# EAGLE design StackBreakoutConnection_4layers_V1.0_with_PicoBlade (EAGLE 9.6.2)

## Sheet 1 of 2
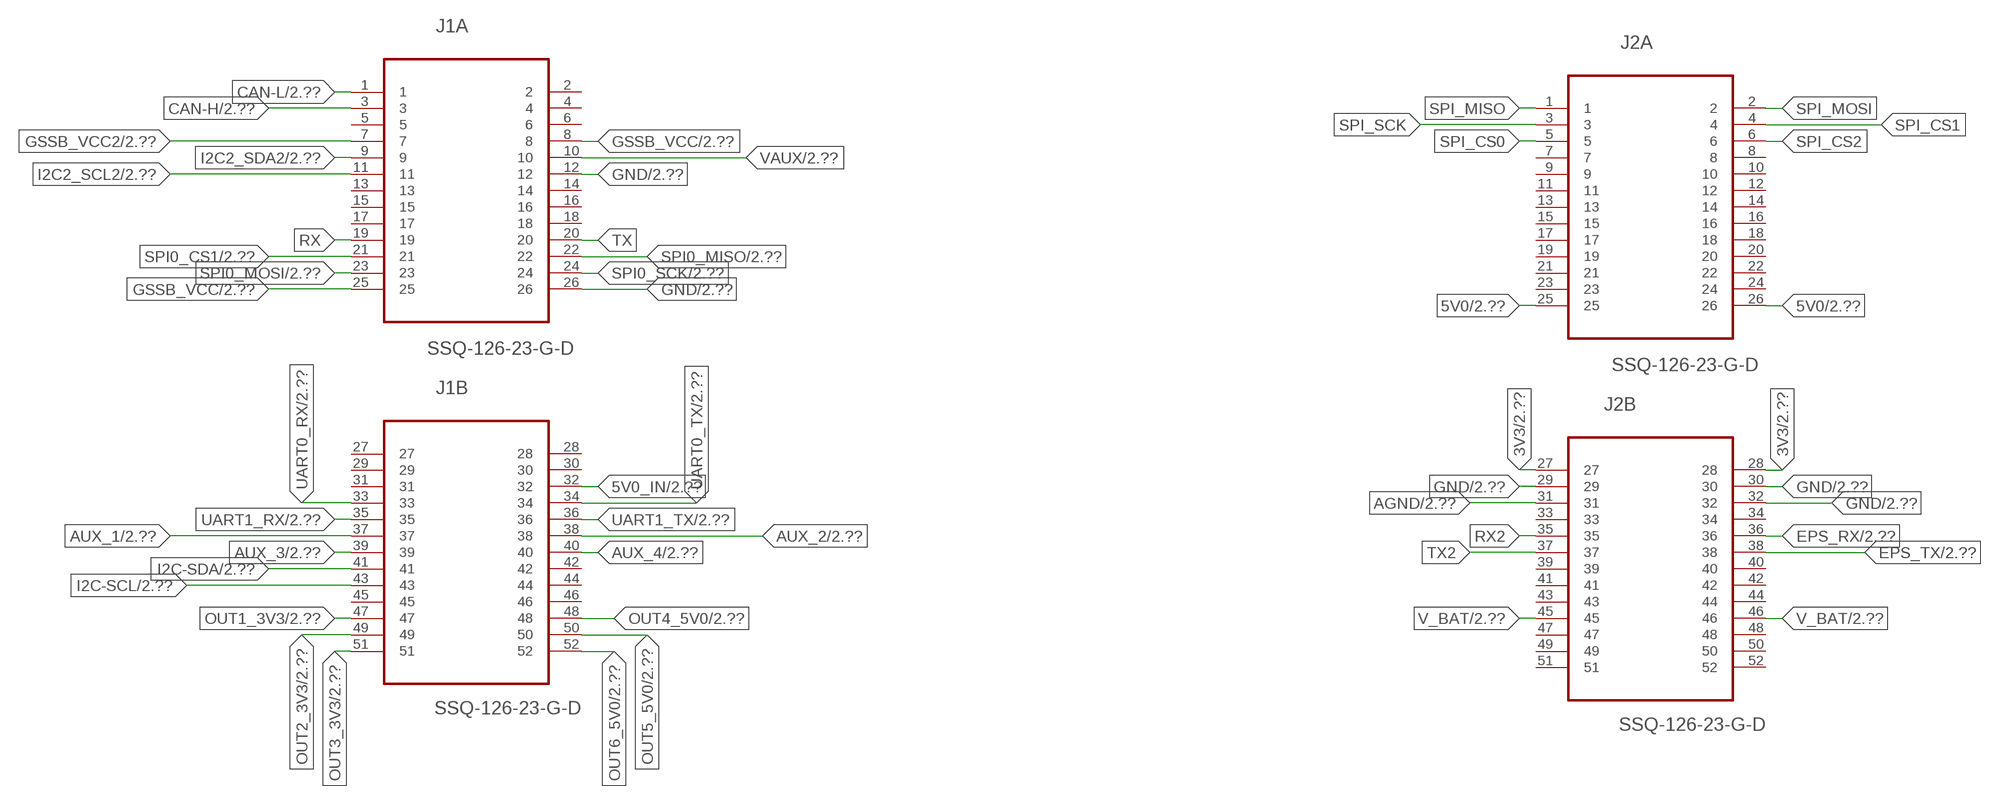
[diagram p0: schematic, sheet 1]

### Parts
J1  SSQ-126-23-G-D  [SAMTEC_SSQ-126-23-G-D]
J2  SSQ-126-23-G-D  [SAMTEC_SSQ-126-23-G-D]

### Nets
3V3: J2.27 J2.28 ; also sheet 2
5V0: J2.25 J2.26 ; also sheet 2
5V0_IN: J1.32 ; also sheet 2
AGND: J2.31 ; also sheet 2
AUX_1: J1.37 ; also sheet 2
AUX_2: J1.38 ; also sheet 2
AUX_3: J1.39 ; also sheet 2
AUX_4: J1.40 ; also sheet 2
CAN-H: J1.3 ; also sheet 2
CAN-L: J1.1 ; also sheet 2
EPS_RX: J2.36 ; also sheet 2
EPS_TX: J2.38 ; also sheet 2
GND: J1.12 J1.26 J2.29 J2.30 J2.32 ; also sheet 2
GSSB_VCC: J1.8 J1.25 ; also sheet 2
GSSB_VCC2: J1.7 ; also sheet 2
I2C2_SCL2: J1.11 ; also sheet 2
I2C2_SDA2: J1.9 ; also sheet 2
I2C-SCL: J1.43 ; also sheet 2
I2C-SDA: J1.41 ; also sheet 2
OUT1_3V3: J1.47 ; also sheet 2
OUT2_3V3: J1.49 ; also sheet 2
OUT3_3V3: J1.51 ; also sheet 2
OUT4_5V0: J1.48 ; also sheet 2
OUT5_5V0: J1.50 ; also sheet 2
OUT6_5V0: J1.52 ; also sheet 2
RX: J1.19
RX2: J2.35
SPI0_CS1: J1.21 ; also sheet 2
SPI0_MISO: J1.22 ; also sheet 2
SPI0_MOSI: J1.23 ; also sheet 2
SPI0_SCK: J1.24 ; also sheet 2
SPI_CS0: J2.5
SPI_CS1: J2.4
SPI_CS2: J2.6
SPI_MISO: J2.1
SPI_MOSI: J2.2
SPI_SCK: J2.3
TX: J1.20
TX2: J2.37
UART0_RX: J1.33 ; also sheet 2
UART0_TX: J1.34 ; also sheet 2
UART1_RX: J1.35 ; also sheet 2
UART1_TX: J1.36 ; also sheet 2
V_BAT: J2.45 J2.46 ; also sheet 2
VAUX: J1.10 ; also sheet 2
Unconnected: J1.2 J1.4 J1.5 J1.6 J1.13 J1.14 J1.15 J1.16 J1.17 J1.18 J1.27 J1.28 J1.29 J1.30 J1.31 J1.42 J1.44 J1.45 J1.46 J2.7 J2.8 J2.9 J2.10 J2.11 J2.12 J2.13 J2.14 J2.15 J2.16 J2.17 J2.18 J2.19 J2.20 J2.21 J2.22 J2.23 J2.24 J2.33 J2.34 J2.39 J2.40 J2.41 J2.42 J2.43 J2.44 J2.47 J2.48 J2.49 J2.50 J2.51 J2.52

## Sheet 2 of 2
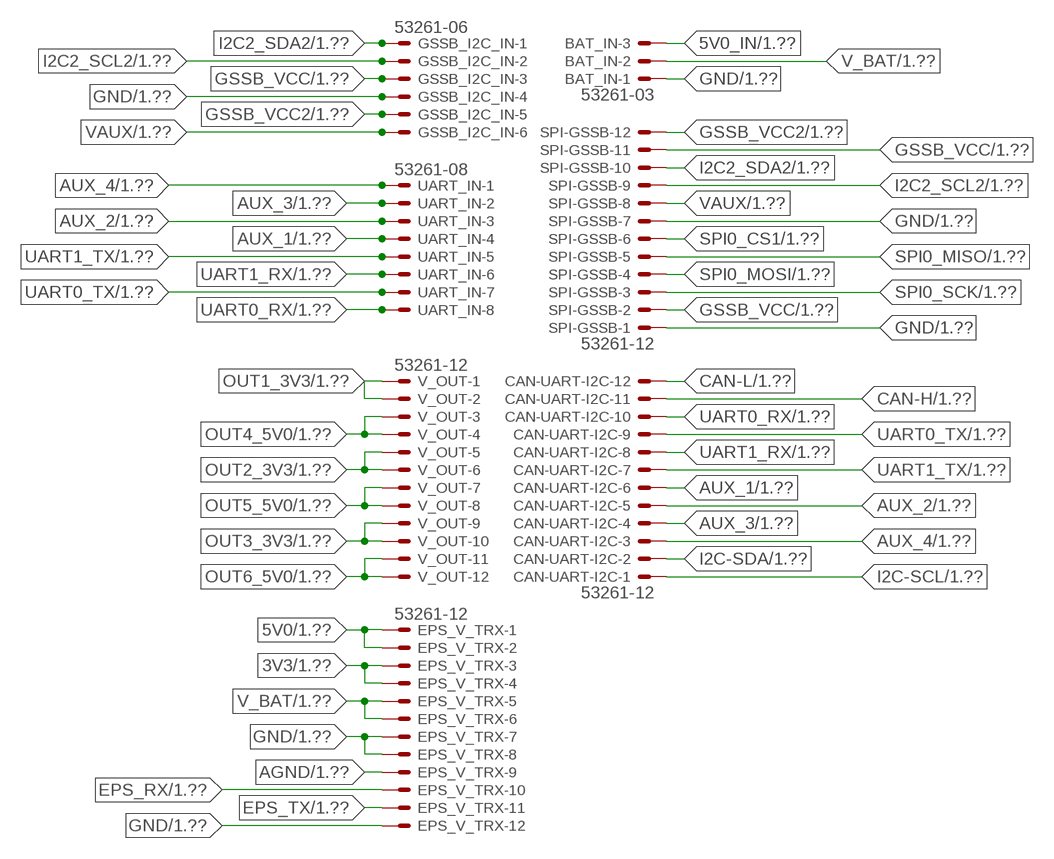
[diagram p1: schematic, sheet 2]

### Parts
BAT_IN  53261-03  [53261-03]
CAN-UART-I2C  53261-12  [53261-12]
EPS_V_TRX  53261-12  [53261-12]
GSSB_I2C_IN  53261-06  [53261-06]
SPI-GSSB  53261-12  [53261-12]
UART_IN  53261-08  [53261-08]
V_OUT  53261-12  [53261-12]

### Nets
3V3: EPS_V_TRX.3 EPS_V_TRX.4 ; also sheet 1
5V0: EPS_V_TRX.1 EPS_V_TRX.2 ; also sheet 1
5V0_IN: BAT_IN.3 ; also sheet 1
AGND: EPS_V_TRX.9 ; also sheet 1
AUX_1: CAN-UART-I2C.6 UART_IN.4 ; also sheet 1
AUX_2: CAN-UART-I2C.5 UART_IN.3 ; also sheet 1
AUX_3: CAN-UART-I2C.4 UART_IN.2 ; also sheet 1
AUX_4: CAN-UART-I2C.3 UART_IN.1 ; also sheet 1
CAN-H: CAN-UART-I2C.11 ; also sheet 1
CAN-L: CAN-UART-I2C.12 ; also sheet 1
EPS_RX: EPS_V_TRX.10 ; also sheet 1
EPS_TX: EPS_V_TRX.11 ; also sheet 1
GND: BAT_IN.1 EPS_V_TRX.7 EPS_V_TRX.8 EPS_V_TRX.12 GSSB_I2C_IN.4 SPI-GSSB.1 SPI-GSSB.7 ; also sheet 1
GSSB_VCC: GSSB_I2C_IN.3 SPI-GSSB.2 SPI-GSSB.11 ; also sheet 1
GSSB_VCC2: GSSB_I2C_IN.5 SPI-GSSB.12 ; also sheet 1
I2C2_SCL2: GSSB_I2C_IN.2 SPI-GSSB.9 ; also sheet 1
I2C2_SDA2: GSSB_I2C_IN.1 SPI-GSSB.10 ; also sheet 1
I2C-SCL: CAN-UART-I2C.1 ; also sheet 1
I2C-SDA: CAN-UART-I2C.2 ; also sheet 1
OUT1_3V3: V_OUT.1 V_OUT.2 ; also sheet 1
OUT2_3V3: V_OUT.5 V_OUT.6 ; also sheet 1
OUT3_3V3: V_OUT.9 V_OUT.10 ; also sheet 1
OUT4_5V0: V_OUT.3 V_OUT.4 ; also sheet 1
OUT5_5V0: V_OUT.7 V_OUT.8 ; also sheet 1
OUT6_5V0: V_OUT.11 V_OUT.12 ; also sheet 1
SPI0_CS1: SPI-GSSB.6 ; also sheet 1
SPI0_MISO: SPI-GSSB.5 ; also sheet 1
SPI0_MOSI: SPI-GSSB.4 ; also sheet 1
SPI0_SCK: SPI-GSSB.3 ; also sheet 1
UART0_RX: CAN-UART-I2C.10 UART_IN.8 ; also sheet 1
UART0_TX: CAN-UART-I2C.9 UART_IN.7 ; also sheet 1
UART1_RX: CAN-UART-I2C.8 UART_IN.6 ; also sheet 1
UART1_TX: CAN-UART-I2C.7 UART_IN.5 ; also sheet 1
V_BAT: BAT_IN.2 EPS_V_TRX.5 EPS_V_TRX.6 ; also sheet 1
VAUX: GSSB_I2C_IN.6 SPI-GSSB.8 ; also sheet 1

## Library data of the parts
BAT_IN = con-molex:53?-03: CONNECTOR wire to board 1.25 mm (.049 inch) pitch header; MF: MOLEX; MPN: 53261-0390; OC_FARNELL: 1125359; OC_NEWARK: 57H5006
CAN-UART-I2C EPS_V_TRX SPI-GSSB V_OUT = con-molex:53?-12: CONNECTOR wire to board 1.25 mm (.049 inch) pitch header; MF: MOLEX; MPN: 53261-1271; OC_FARNELL: 1125363; OC_NEWARK: 59J0244
GSSB_I2C_IN = con-molex:53?-06: CONNECTOR wire to board 1.25 mm (.049 inch) pitch header; MF: MOLEX; OC_FARNELL: 1125375; OC_NEWARK: unknown
J1 J2 = SPEL:SSQ-126-23-G-D: CONN RECEPTACLE, 2.54MM, DUAL, 52WAY; MPN: SSQ-126-23-G-D; OC_FARNELL: -; OC_NEWARK: 82P0504; PACKAGE: RECEPTACLE, 2.54MM, DUAL, 52WAY; SUPPLIER: Samtec
UART_IN = con-molex:53?-08: CONNECTOR wire to board 1.25 mm (.049 inch) pitch header; MF: MOLEX; OC_FARNELL: 1125376; OC_NEWARK: unknown

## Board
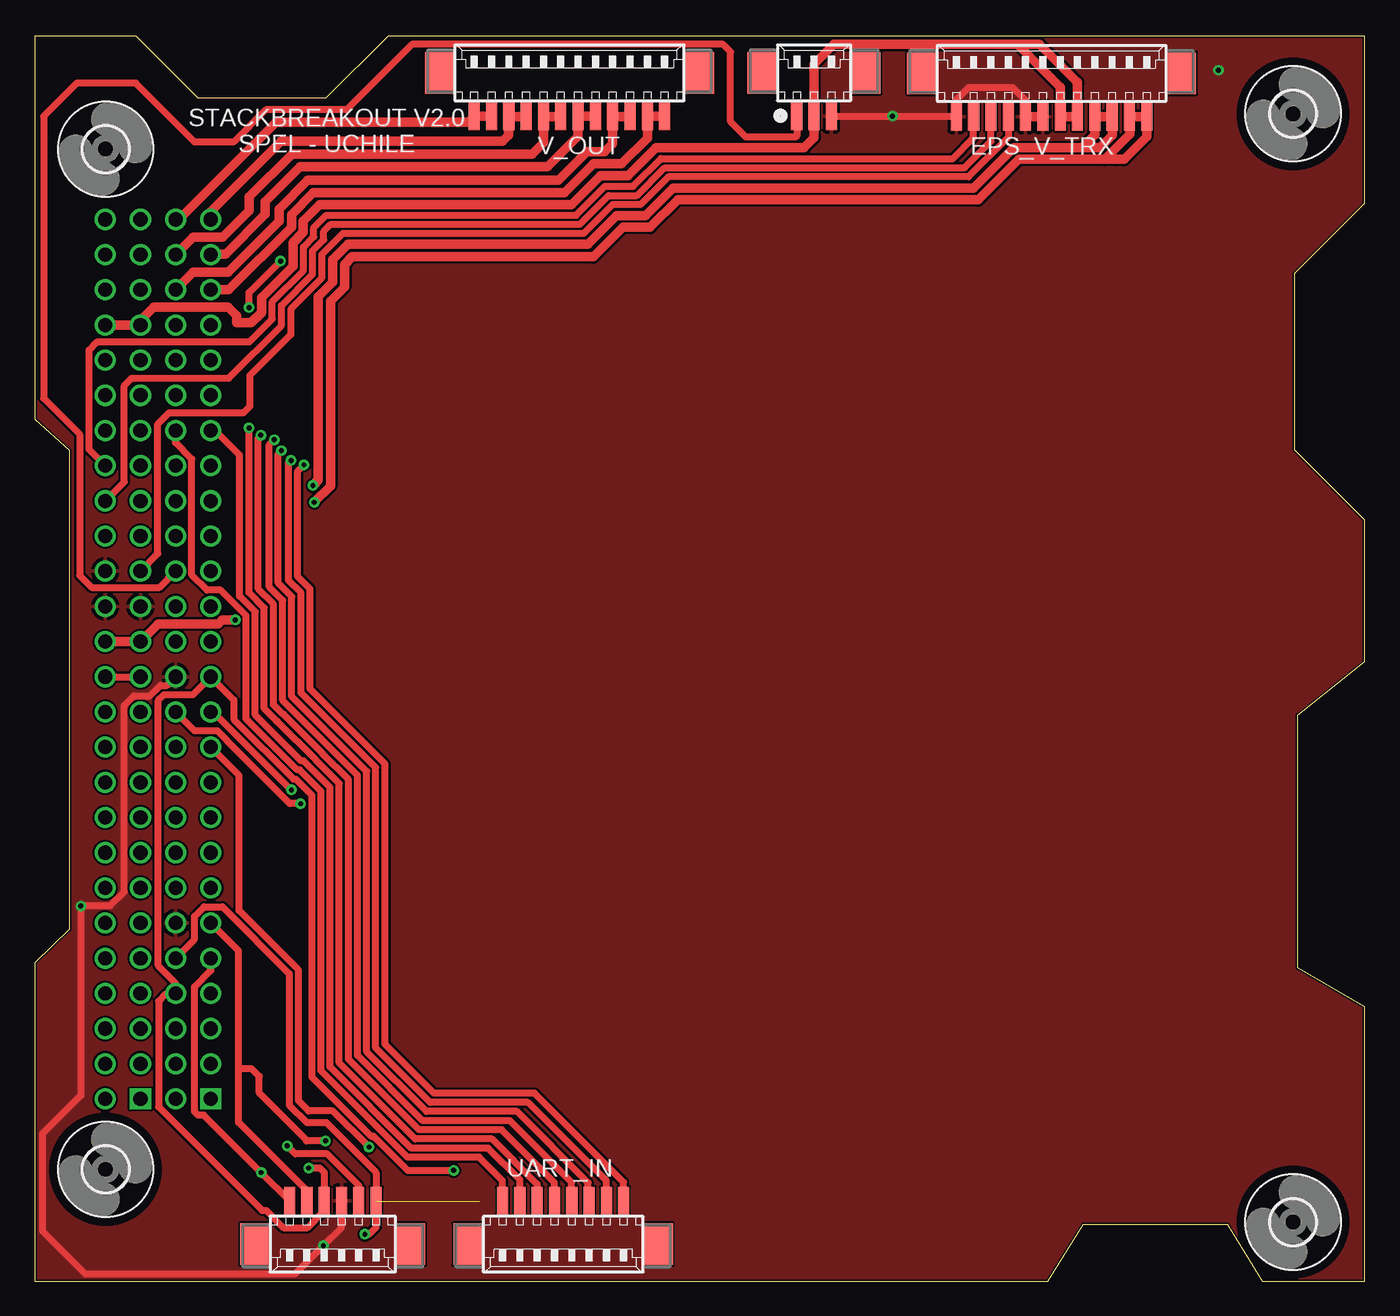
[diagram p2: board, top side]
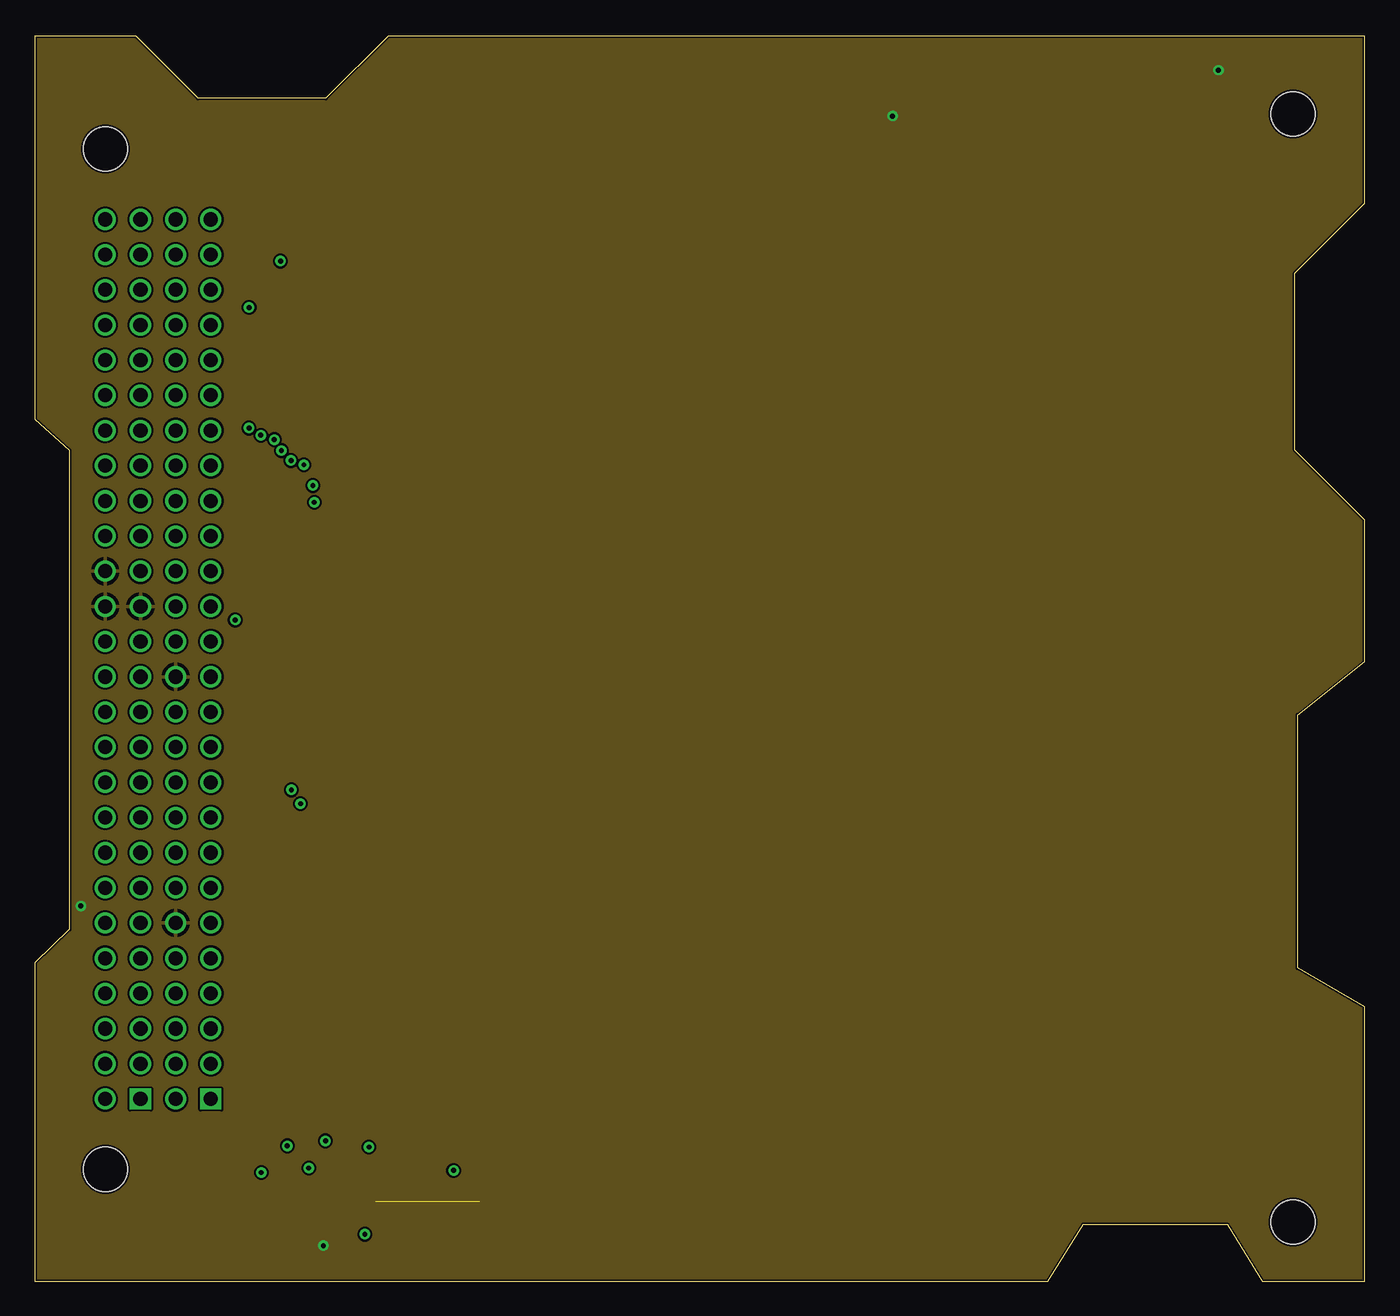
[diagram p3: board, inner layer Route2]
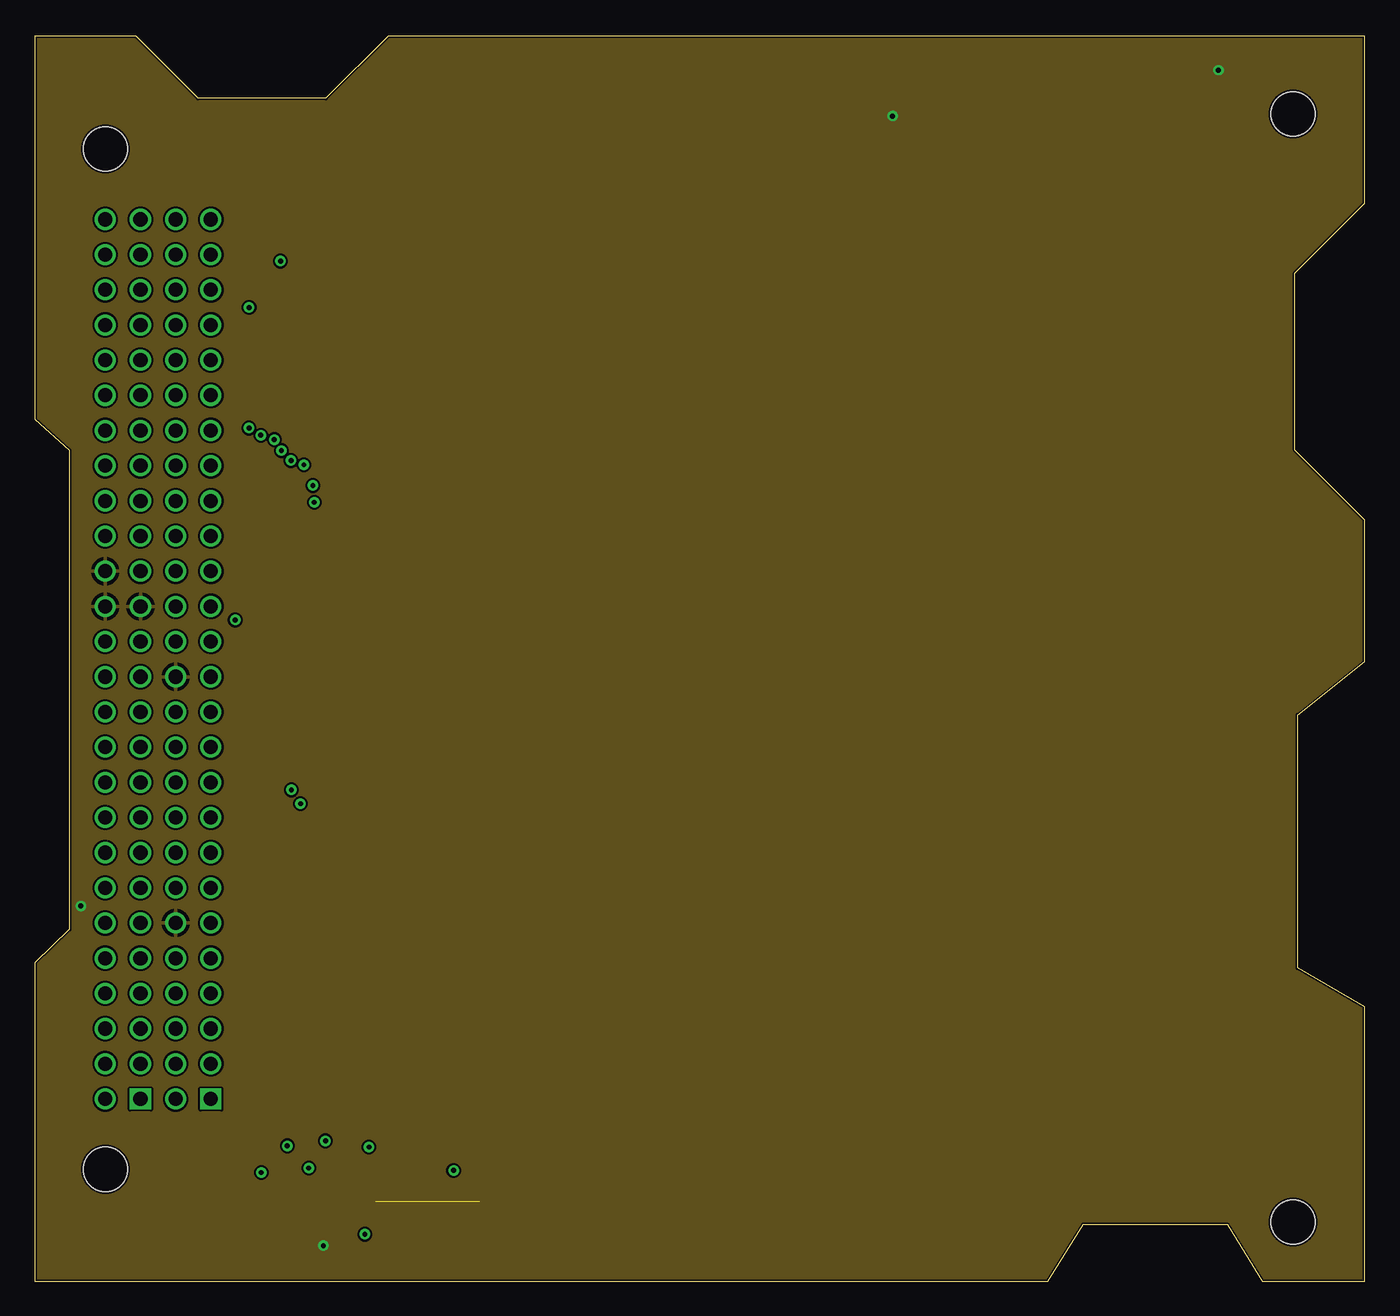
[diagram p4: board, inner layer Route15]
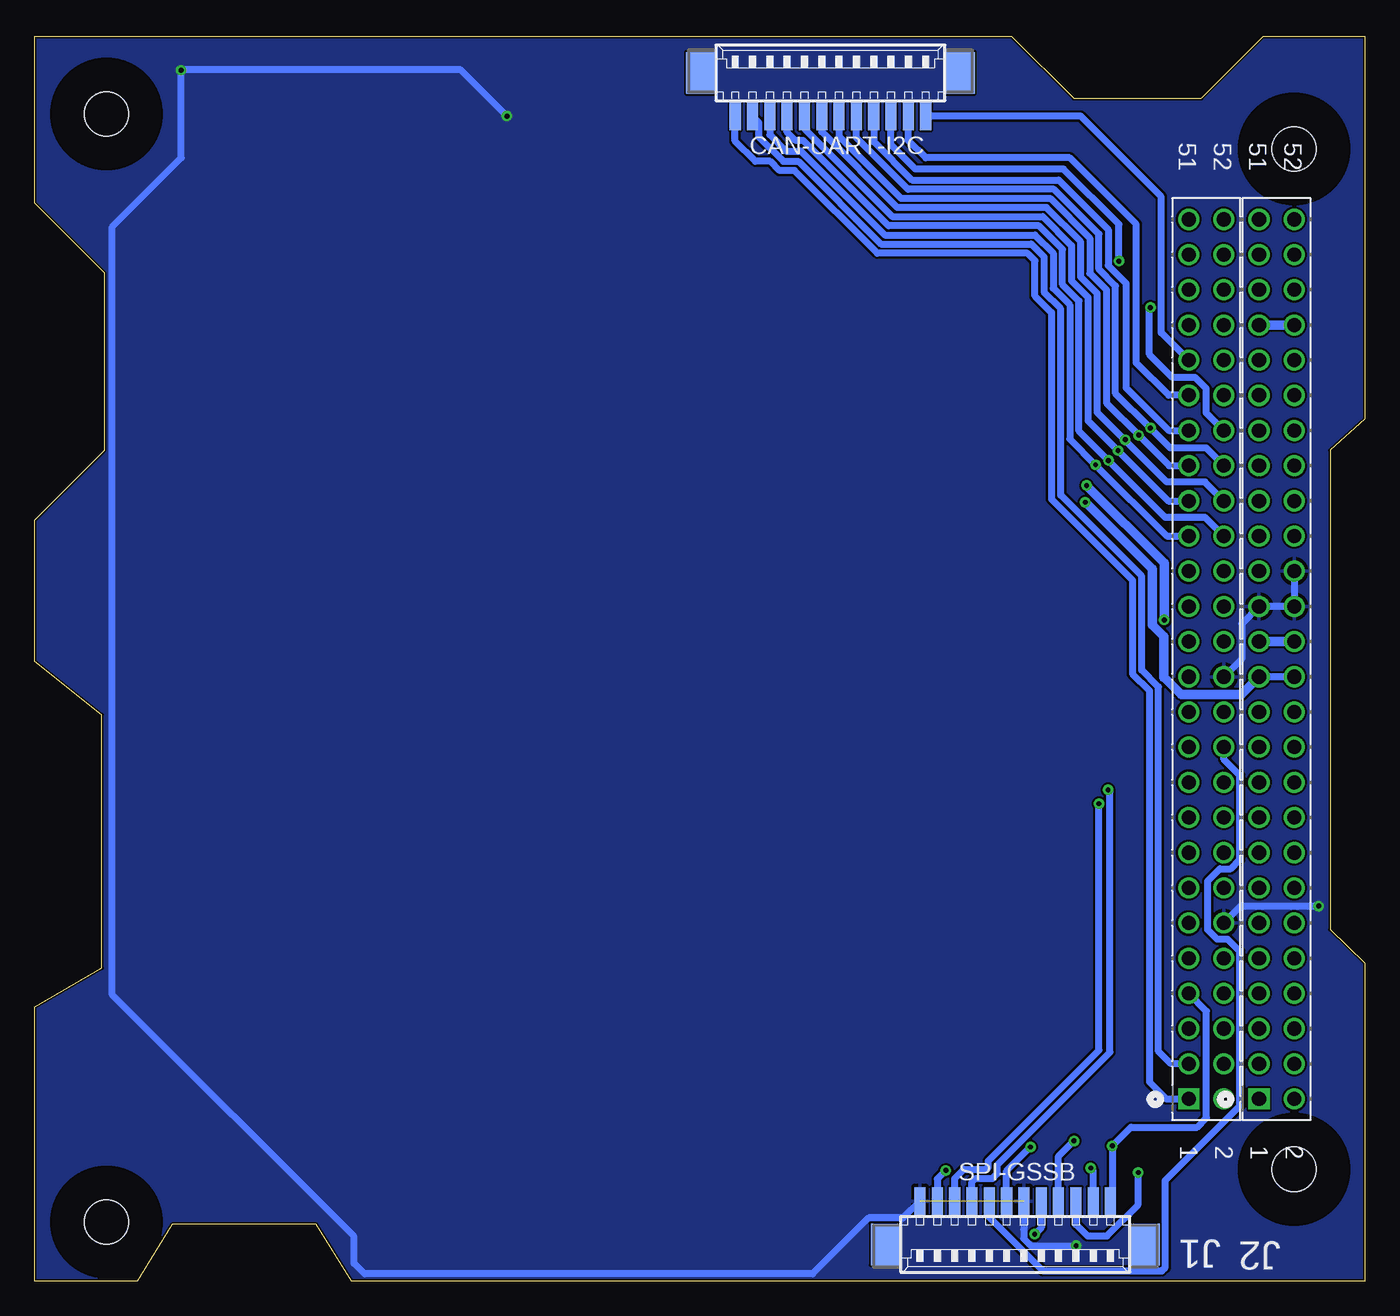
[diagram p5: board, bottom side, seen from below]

Size 96.04 x 89.88 mm. Coordinates in mm from the lower left corner, seen from the top.
Outline: 90.98,72.77 96.04,77.83 96.04,89.88 25.51,89.88 21.02,85.4 11.8,85.4 7.32,89.88 0,89.88 0,62.23 2.5,60 2.5,25.4 0,23 0,0 73.15,0 75.7,4.1 86.09,4.1 88.65,0 96.01,0 96.01,19.81 91.19,22.61 91.19,40.89 96.04,44.76 96.04,54.97 90.98,60.02 90.98,72.77
Copper layers (1+2*15+16): Top 0.035mm / dielectric 1.5mm / Route2 0.035mm / dielectric 0.15mm / Route15 0.035mm / dielectric 0.2mm / Bottom 0.035mm
Design rules "default *": minimum track width 20mil, minimum drill 0.2mm, track to track 6mil, track to pad 6mil, pad to pad 6mil, via to via 6mil, smd to smd 6mil, copper to edge 6mil, drill to drill 6mil, minimum pad ring 10mil, minimum via ring 8mil, stop-mask expansion 4mil, vias tented up to drill 0mil, thermal gap 10mil

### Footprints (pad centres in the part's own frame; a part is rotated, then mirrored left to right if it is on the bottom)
53261-03 = smd 0.8 x 2: 1 1.25,-2.5; 2 0,-2.5; 3 -1.25,-2.5 | smd 2.1 x 3: S1 3.75,0.625; S2 -3.75,0.625
53261-12 = smd 0.8 x 2: 1 6.875,-2.5; 2 5.625,-2.5; 3 4.375,-2.5; 4 3.125,-2.5; 5 1.875,-2.5; 6 0.625,-2.5; 7 -0.625,-2.5; 8 -1.875,-2.5; 9 -3.125,-2.5; 10 -4.375,-2.5; 11 -5.625,-2.5; 12 -6.875,-2.5 | smd 2.1 x 3: S1 9.375,0.625; S2 -9.375,0.625
3,2 = hole 3.2: 0,0
53261-06 = smd 0.8 x 2: 1 3.125,-2.5; 2 1.875,-2.5; 3 0.625,-2.5; 4 -0.625,-2.5; 5 -1.875,-2.5; 6 -3.125,-2.5 | smd 2.1 x 3: S1 5.625,0.625; S2 -5.625,0.625
SAMTEC_SSQ-126-23-G-D = drill 1.016 square: 1 63.5,-2.54 | drill 1.016: 2 63.5,0; 3 60.96,-2.54; 4 60.96,0; 5 58.42,-2.54; 6 58.42,0; 7 55.88,-2.54; 8 55.88,0; 9 53.34,-2.54; 10 53.34,0; 11 50.8,-2.54; 12 50.8,0; 13 48.26,-2.54; 14 48.26,0; 15 45.72,-2.54; 16 45.72,0; 17 43.18,-2.54; 18 43.18,0; 19 40.64,-2.54; 20 40.64,0; 21 38.1,-2.54; 22 38.1,0; 23 35.56,-2.54; 24 35.56,0; 25 33.02,-2.54; 26 33.02,0; 27 30.48,-2.54; 28 30.48,0; 29 27.94,-2.54; 30 27.94,0; 31 25.4,-2.54; 32 25.4,0; 33 22.86,-2.54; 34 22.86,0; 35 20.32,-2.54; 36 20.32,0; 37 17.78,-2.54; 38 17.78,0; 39 15.24,-2.54; 40 15.24,0; 41 12.7,-2.54; 42 12.7,0; 43 10.16,-2.54; 44 10.16,0; 45 7.62,-2.54; 46 7.62,0; 47 5.08,-2.54; 48 5.08,0; 49 2.54,-2.54; 50 2.54,0; 51 0,-2.54; 52 0,0
53261-08 = smd 0.8 x 2: 1 4.375,-2.5; 2 3.125,-2.5; 3 1.875,-2.5; 4 0.625,-2.5; 5 -0.625,-2.5; 6 -1.875,-2.5; 7 -3.125,-2.5; 8 -4.375,-2.5 | smd 2.1 x 3: S1 6.875,0.625; S2 -6.875,0.625

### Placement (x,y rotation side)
BAT_IN  56.27,86.62 0 top
CAN-UART-I2C  38.58,86.62 0 bottom
EPS_V_TRX  73.42,86.58 0 top
GND  [3,2]  90.85,4.27 0 top
GSSB_I2C_IN  21.53,3.3 180 top
J1  10.18,76.66 270 bottom
J2  5.1,76.66 270 bottom
SPI-GSSB  25.24,3.28 180 bottom
U$1  [3,2]  5.12,81.74 0 top
U$2  [3,2]  90.85,84.28 0 top
U$4  [3,2]  5.12,8.08 0 top
UART_IN  38.16,3.3 180 top
V_OUT  38.61,86.61 0 top

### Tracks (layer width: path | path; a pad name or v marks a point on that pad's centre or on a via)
3V3  (via drill 0.35)
  Top 0.7: J2.28 J2.27 | J2.27 7.82,46.18 | 75.6,81.85 70.7,81.85 67.78,78.93 46.08,78.93 44.09,76.94 42.03,76.94 39.96,74.87 22.64,74.87 21.52,73.76 21.52,72.13 20.48,71.09 20.48,57.84 v20.09,57.45 | 75.6,81.85 76.54,82.79 EPS_V_TRX.4 EPS_V_TRX.3 77.79,82.74 76.9,81.85 75.6,81.85 | v14.48,47.74 13.53,47.74 13.24,47.46 8.92,47.46 J2.27
  Bottom 0.7: J2.28 J2.27 | v20.09,57.45 14.48,51.84 v14.48,47.74
5V0  (via drill 0.35)
  Top 0.508: J2.26 J2.25
  Top 0.7: 77.25,81 79.06,82.81 79.06,84.05 EPS_V_TRX.2 EPS_V_TRX.1 80.29,82.63 78.66,81 78.03,81 77.25,81 | 77.25,81 71.06,81 68.14,78.08 46.43,78.08 44.44,76.09 42.47,76.09 40.34,73.96 22.93,73.96 22.37,73.4 22.37,71.77 21.35,70.75 21.35,57.4 v20.19,56.24
  Bottom 0.508: J2.26 J2.25
  Bottom 0.7: v20.19,56.24 15.36,51.41 15.36,47.38 14.52,46.53 14.52,43.6 14.47,43.6 13.24,42.38 8.9,42.38 J2.25
5V0_IN
  Top 0.508: BAT_IN.3 55.02,82.67 54.95,82.6 51.35,82.6 50.25,83.7 50.25,88.75 49.7,89.3 27.25,89.3 22.52,84.57 16.68,84.57 14.36,82.25 11.55,82.25 7.3,86.5 3.05,86.5 0.65,84.1 0.65,63.75 3.25,61.15 3.25,50.95 4.11,50.09 9.01,50.09 J1.32
AGND
  Top 0.508: EPS_V_TRX.9 70.29,82.59 67.43,79.73 45.76,79.73 43.76,77.73 41.72,77.73 39.63,75.64 22.25,75.64 20.73,74.12 20.73,72.42 18.49,70.18 18.49,68.34 15.56,65.41 15.56,63.18 15.08,62.7 9.7,62.7 8.9,61.9 8.9,52.52 J2.31
AUX_1  (via drill 0.35)
  Top 0.508: UART_IN.4 37.53,7.12 33.72,10.93 27.74,10.93 22.65,16.02 22.65,36.21 20.79,38.07 20.79,38.12 17.99,40.92 17.94,40.92 17.25,41.62 17.25,48.89 16.14,49.99 16.14,60.89 v16.33,61.08
  Bottom 0.508: CAN-UART-I2C.6 37.96,82.66 33.48,78.18 22.71,78.18 19.86,75.32 19.86,72.78 18.66,71.58 18.66,63.41 v16.33,61.08 14.13,58.88 J1.37
AUX_2  (via drill 0.35)
  Top 0.508: UART_IN.3 36.29,7.01 33.02,10.27 27.47,10.27 21.99,15.75 21.99,35.92 20.31,37.61 20.31,37.62 17.51,40.42 | 17.51,40.42 17.47,40.42 | 17.51,40.42 16.59,41.34 16.59,48.61 15.48,49.72 v15.48,61.6
  Bottom 0.508: J1.38 11.45,60.15 14.05,60.15 15.48,61.58 | 15.48,61.58 18,64.1 18,71.86 19.2,73.05 19.2,75.59 22.44,78.84 32.97,78.84 36.71,82.57 CAN-UART-I2C.5 | v15.48,61.6 15.48,61.58
AUX_3
  Top 0.508: UART_IN.2 35.03,7.33 32.75,9.61 27.2,9.61 21.33,15.48 21.33,35.65 19.41,37.58 19.23,37.58 15.93,40.88 15.93,48.34 14.8,49.46 14.8,59.65 13.03,61.42 J1.39
  Bottom 0.508: CAN-UART-I2C.4 35.46,82.26 32.7,79.5 22.1,79.5 18.54,75.94 18.54,73.33 17.25,72.04 17.25,64.5 14.17,61.42 J1.39
AUX_4  (via drill 0.35)
  Top 0.508: v15.48,70.3 15.48,71.39 v17.75,73.65 | UART_IN.1 33.78,7.26 32.09,8.95 26.92,8.95 20.67,15.2 20.67,35.38 19.13,36.91 18.96,36.91 15.27,40.61 15.27,48.06 13.44,49.89 12.44,49.89 11.35,50.98 11.35,59.36 10.18,60.53 J1.40
  Bottom 0.508: J1.40 11.45,62.69 11.45,64.45 12.25,65.25 13.9,65.25 15.55,66.9 15.55,70.23 v15.48,70.3 | v17.75,73.65 17.75,76.3 21.75,80.3 32.45,80.3 34.21,82.06 CAN-UART-I2C.3
CAN-H
  Bottom 0.508: CAN-UART-I2C.11 43.77,83.67 43.77,82.63 41.98,80.85 40.9,80.85 34.93,74.88 24.08,74.88 23.16,73.95 23.16,71.41 21.96,70.22 21.96,56.74 16.12,50.9 16.12,44.13 14.9,42.91 14.9,16.6 14,15.7 J1.3
CAN-L
  Bottom 0.508: CAN-UART-I2C.12 45.46,82.31 44,80.85 42.92,80.85 42.26,80.19 41.17,80.19 35.2,74.22 24.35,74.22 23.82,73.68 23.82,71.14 22.62,69.94 22.62,56.47 16.78,50.62 16.78,43.85 15.56,42.64 15.56,14.39 14.32,13.15 J1.1
EPS_RX
  Top 0.508: J2.36 6.47,57.71 6.47,64.67 7,65.2 14.02,65.2 17.82,69 17.82,70.44 20.07,72.69 20.07,74.39 20.87,75.19 20.87,75.8 21.37,76.3 39.36,76.3 41.45,78.39 43.48,78.39 45.48,80.39 67.14,80.39 69.04,82.29 EPS_V_TRX.10
EPS_TX
  Top 0.508: EPS_V_TRX.11 67.79,82.54 66.3,81.05 45.21,81.05 43.21,79.05 41.18,79.05 39.09,76.96 21.05,76.96 20.16,76.07 20.16,75.41 19.41,74.67 19.41,72.97 17.15,70.71 17.15,69.47 15.52,67.83 4.53,67.83 3.93,67.23 3.93,60.05 J2.38
GND  (via drill 0.35)  (1 unrouted)
  Top 0.508: BAT_IN.1 v61.94,84.12 66.5,84.12 EPS_V_TRX.12 66.54,85.29 67.45,86.2 70.6,86.2 71.54,85.26 EPS_V_TRX.8 | J1.26 9.56,43.02 9.07,43.02 8.31,42.27 7.16,42.27 6.47,41.58 6.47,28.12 5.47,27.12 3.33,27.12 v3.33,27.09 3.33,13.42 0.56,10.65 0.56,3.63 3.67,0.52 18.8,0.52 v20.84,2.56 22.15,3.87 GSSB_I2C_IN.4
  Top 0.7: EPS_V_TRX.8 EPS_V_TRX.7
  Bottom 0.508: J2.32 J2.30 J2.29 8.9,47.46 8.9,44.92 J1.26 | v61.94,84.12 65.27,87.45 85.44,87.45 | 85.44,87.45 v85.46,87.43 | J1.12 8.96,27.08 3.66,27.08 3.65,27.09 v3.33,27.09 | v20.84,2.56 24.12,2.56 24.62,3.06 24.62,3.71 24.61,3.73 SPI-GSSB.7 | 32.1,5.77 SPI-GSSB.1 33.33,4.56 35.83,4.56 39.88,0.52 72.21,0.52 72.98,1.29 72.98,3.23 90.42,20.67 90.42,76.13 85.44,81.11 85.44,87.45
  pour Route15: -0.22,90.12 7.77,90.12 7.77,90.04 12.04,85.77 20.96,85.77 26.02,90.83 96.4,90.83 96.71,90.52 96.71,77.77 91.45,72.52 91.45,60.39 96.5,55.34 96.5,44.84 91.56,39.9 91.56,22.84 96.45,20.03 96.45,-0.36 88.28,-0.36 85.72,3.61 76.26,3.61 73.9,-0.36 -0.35,-0.36 -0.35,23.1 2.23,25.67 2.23,59.72 -0.23,62.18 -0.23,90.12 -0.23,90.12
  pour Top: -0.25,-0.13 73.41,-0.13 76.03,3.81 85.89,3.81 88.6,-0.25 96.27,-0.25 96.27,20.57 91.44,22.99 91.44,40.58 96.27,44.2 96.27,55.24 91.31,60.2 91.31,72.64 96.39,77.72 96.39,90.17 24.89,90.17 20.57,85.85 11.65,85.85 8.22,90.42 -0.25,90.42 -0.25,62.23 2.29,59.69 2.29,25.65 -0.25,23.11
  pour Route2: -0.46,-0.28 73.46,-0.28 76.08,3.66 85.9,3.66 88.53,-0.28 96.32,-0.28 96.32,20.42 91.87,22.64 91.87,40.87 96.32,44.2 96.32,55.22 91.36,60.17 91.36,72.62 96.44,77.7 96.44,90.4 25.32,90.4 20.75,85.83 11.77,85.83 8.62,90.02 -0.2,90.02 -0.2,62.33 2.08,60.05 2.08,25.88 -0.46,23.34
  pour Bottom: -0.27,90.34 7.08,90.34 7.08,90.4 11.74,85.74 11.74,85.86 20.77,85.86 26.09,91.18 95.59,91.18 96.65,90.11 96.65,77.24 91.53,72.11 91.53,60.11 96.71,54.93 96.71,44.56 91.64,39.49 91.64,22.93 96.27,20.25 96.27,-0.51 88.48,-0.51 85.92,3.45 76.54,3.45 74.18,-0.51 -0.4,-0.51 -0.4,23.33 2.18,25.9 2.18,59.57 -0.28,62.03 -0.28,90.35 -0.28,90.35
GSSB_VCC  (via drill 0.35)
  Top 0.508: v19.79,8.17 20.59,8.17 20.9,7.86 GSSB_I2C_IN.3 20.9,5.08 19.7,3.87 17.96,3.87 16.72,5.11 16.41,5.11 8.94,12.58 8.94,20.21 9.51,20.78 J1.8 10.18,21.52 8.93,22.77 8.93,41.95 9.34,42.36 11.44,42.36 J1.25 14.38,41.98 14.38,40.56 18.68,36.26 18.86,36.26 20.01,35.1 20.01,14.75 24.29,10.47 24.46,10.47 26.94,8 v30.25,8
  Bottom 0.508: SPI-GSSB.11 19.61,8 v19.79,8.17 | v30.25,8 30.86,7.38 SPI-GSSB.2
GSSB_VCC2  (via drill 0.35)
  Top 0.508: GSSB_I2C_IN.5 23.4,6.91 21.12,9.19 18.82,9.19 v18.24,9.77
  Bottom 0.508: v18.24,9.77 18.36,9.65 | 18.36,5.79 SPI-GSSB.12 18.24,5.91 v18.24,9.77 | v18.24,9.77 16.89,11.12 12.11,11.12 11.43,11.8 11.43,19.49 J1.7
I2C2_SCL2  (via drill 0.35)
  Top 0.508: GSSB_I2C_IN.2 19.66,6.52 14.72,11.46 14.72,15.35 | J1.11 14.72,23.86 14.72,15.35 | v21,10.13 19.63,10.13 19.65,10.15 16.21,13.6 16.21,14.8 15.66,15.35 14.72,15.35
  Bottom 0.508: SPI-GSSB.9 22.11,9.02 v21,10.13
I2C2_SDA2  (via drill 0.35)
  Top 0.508: J1.9 12.72,22.43 11.55,21.26 11.55,12.23 11.79,11.99 12.21,11.99 v16.36,7.84 GSSB_I2C_IN.1
  Bottom 0.508: SPI-GSSB.10 20.86,4.11 20.03,3.27 18.62,3.27 16.36,5.53 v16.36,7.84
I2C-SCL
  Bottom 0.508: J1.43 14.7,68.48 14.7,78.3 20.52,84.12 CAN-UART-I2C.1
I2C-SDA
  Bottom 0.508: J1.41 14.16,63.96 16.5,66.3 16.5,76.3 21.3,81.1 31.7,81.1 32.96,82.36 CAN-UART-I2C.2
OUT1_3V3
  Top 0.7: J1.47 14.02,71.58 18.54,76.1 18.54,77.01 20.11,78.58 38.25,78.58 40.34,80.67 42.37,80.67 44.23,82.53 V_OUT.2 V_OUT.1
OUT2_3V3
  Top 0.508: J1.49 12.77,74.17
  Top 0.7: 12.77,74.17 13.78,74.17 16.65,77.03 16.65,77.92 19.17,80.45 37.01,80.45 39.23,82.67 V_OUT.6 V_OUT.5
OUT3_3V3
  Top 0.508: 34.23,84.07 V_OUT.10 | V_OUT.9 35.44,84.07
  Top 0.7: J1.51 12.72,77.2 17.82,82.3 33.78,82.3 34.23,82.75 34.23,84.07 35.44,84.07
OUT4_5V0
  Top 0.508: 41.73,84.07 V_OUT.4 | V_OUT.3 42.94,84.07
  Top 0.7: J1.48 11.45,72.85 13.96,72.85 17.66,76.55 17.66,77.42 19.72,79.48 37.83,79.48 39.88,81.53 41.15,81.53 41.73,82.12 41.73,84.07 42.94,84.07
OUT5_5V0
  Top 0.508: 36.73,84.07 V_OUT.8 | V_OUT.7 37.94,84.07
  Top 0.7: J1.50 11.45,75.39 13.58,75.39 15.49,77.3 15.49,78.29 18.57,81.37 35.9,81.37 36.73,82.2 36.73,84.07 37.94,84.07
OUT6_5V0
  Top 0.7: J1.52 10.44,76.66 17.45,83.66 31.28,83.66 V_OUT.12 V_OUT.11
SPI0_CS1  (via drill 0.35)
  Top 0.508: v24.14,9.69 21.53,12.3 19.78,12.3 19.05,13.03 19.05,22.47 14.76,26.76 14.76,36.52 J1.21
  Bottom 0.508: SPI-GSSB.6 25.86,7.96 v24.14,9.69
SPI0_MISO
  Bottom 0.508: SPI-GSSB.5 27.1,5.77 27.1,4.61 23.24,0.75 14.65,0.75 14.41,0.99 14.41,7.28 9.01,12.68 9.01,23.8 9.9,24.69 10.66,24.69 11.35,25.38 11.35,28.88 10.46,29.77 9.7,29.77 9.01,30.46 9.01,36.5 10.18,37.67 J1.22
SPI0_MOSI  (via drill 0.35)
  Top 0.508: v18.54,35.47 12.9,41.1 J1.23
  Bottom 0.508: SPI-GSSB.4 28.36,7.17 28.11,7.42 26.88,7.42 26.52,7.78 26.52,8.41 18.41,16.53 18.41,35.35 v18.54,35.47
SPI0_SCK  (via drill 0.35)
  Top 0.508: J1.24 11.55,39.73 13.2,39.73 13.89,39.04 13.89,39.01 18.41,34.48 v19.2,34.48
  Bottom 0.508: SPI-GSSB.3 29.61,7.42 28.95,8.08 27.3,8.08 27.19,8.2 27.19,8.69 19.2,16.68 v19.2,34.48
UART0_RX  (via drill 0.35)
  Top 0.508: UART_IN.8 42.53,7.15 36.11,13.57 28.84,13.57 25.29,17.12 25.29,37.35 19.89,42.76 19.89,49.98 18.99,50.88 18.99,58.49 v19.44,58.94
  Bottom 0.508: CAN-UART-I2C.10 42.96,82.76 41.8,81.6 40.72,81.6 34.66,75.54 23.81,75.54 22.5,74.23 22.5,71.68 21.3,70.49 21.3,60.8 v19.44,58.94 14.3,53.8 J1.33
UART0_TX  (via drill 0.35)
  Top 0.508: UART_IN.7 41.28,7.25 35.62,12.91 28.57,12.91 24.63,16.84 24.63,37.08 19.23,42.48 19.23,49.71 18.33,50.6 18.33,59.07 v18.51,59.25
  Bottom 0.508: J1.34 11.53,55.15 14.41,55.15 v18.51,59.25 20.64,61.38 20.64,70.76 21.84,71.96 21.84,74.5 23.53,76.2 34.38,76.2 40.53,82.35 41.1,82.35 41.71,82.96 CAN-UART-I2C.9
UART1_RX  (via drill 0.35)
  Top 0.508: UART_IN.6 39.97,5.86 39.97,7.11 34.83,12.25 28.29,12.25 23.97,16.57 23.97,36.81 18.57,42.21 18.57,49.43 17.6,50.4 17.6,59.75 v17.82,59.97
  Bottom 0.508: CAN-UART-I2C.8 40.46,83.21 34.11,76.86 23.26,76.86 21.18,74.77 21.18,72.23 19.98,71.04 19.98,62.13 v17.82,59.97 14.19,56.34 J1.35
UART1_TX  (via drill 0.35)
  Top 0.508: UART_IN.5 38.78,7.13 34.32,11.59 28.02,11.59 23.31,16.3 23.31,36.53 17.91,41.94 17.91,49.16 16.94,50.13 16.94,60.4 v17.3,60.76
  Bottom 0.508: J1.36 11.55,57.71 14.31,57.71 17.35,60.76 | CAN-UART-I2C.7 39.21,82.97 33.75,77.52 22.99,77.52 20.52,75.05 20.52,72.5 19.32,71.31 19.32,62.73 17.35,60.76 | v17.3,60.76 17.35,60.76
V_BAT
  Top 0.508: J2.45 7.49,69.19
  Top 0.7: 70.95,89.3 57.7,89.3 56.27,87.87 BAT_IN.2 56.27,82.57 55.54,81.84 44.86,81.84 42.84,79.81 40.85,79.81 38.76,77.72 20.57,77.72 19.4,76.55 19.4,75.74 18.65,74.99 18.65,73.29 16.38,71.02 16.38,69.94 15.64,69.2 14.6,69.2 14.6,69.7 13.99,70.31 8.61,70.31 7.49,69.19 | 70.95,89.3 74.04,86.21 EPS_V_TRX.6 EPS_V_TRX.5 75.29,86.56 72.55,89.3 70.95,89.3 | J2.46 J2.45
  Bottom 0.7: J2.46 J2.45
VAUX  (via drill 0.35)
  Top 0.508: J1.10 11.55,24.69 11.55,26.34 12.24,27.03 13.56,27.03 18.39,22.2 18.39,12.71 19.64,11.46 21.05,11.46 24.65,7.86 GSSB_I2C_IN.6 24.65,3.89 24.15,3.39 v23.84,3.39
  Bottom 0.508: SPI-GSSB.8 23.36,3.87 v23.84,3.39

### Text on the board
tPlace: STACKBREAKOUT V2.0 / SPEL - UCHILE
